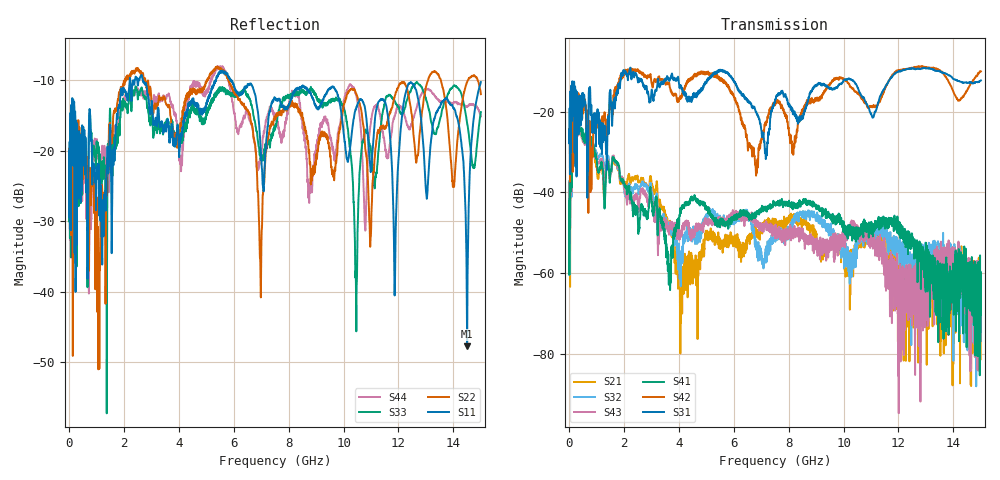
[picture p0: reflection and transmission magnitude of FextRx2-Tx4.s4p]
! FILE: N:\QM 2007\Prüfprotokolle\Highspeed\Konfektionierte Ltg\L45593-D106\D30\8216\0002\Fext\FextRx2-Tx4.s4p
# MHz S DB R 50.00
! FREQ  S11  S12  S13  S14
!  S21  S22  S23  S24
!  S31  S32  S33  S34
!  S41  S42  S43  S44
!  DB  ANG  DB  ANG  DB  ANG  DB  ANG
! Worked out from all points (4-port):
!   2999 points, 10 MHz to 15 GHz, reference 50 ohm
!   strongest paths, dB at 10 MHz, 3.755 GHz, 7.505 GHz, 11.26 GHz, 15 GHz:
!     S31: -24.6, -10.6, -17.4, -17.8, -12.3
!     S42: -24.3, -15.3, -18.5, -18.3, -10.1
!     S41: -42.2, -56.0, -42.7, -46.5, -70.3
!     S43: -48.5, -47.9, -48.9, -55.2, -64.2
!     S32: -41.6, -48.5, -49.1, -50.5, -67.4
!     S21: -49.6, -50.7, -47.5, -51.4, -69.8
!   lowest |S11| = -47.8 dB at 14.5 GHz (marker M1), VSWR 1.01, Z = 49.9 - j0.4 ohm
!   |S11| at or under -10 dB: start of sweep to 2.215 GHz; 2.693 GHz to 5.334 GHz (2.641 GHz wide, 65.8 % of centre); 5.923 GHz to end of sweep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
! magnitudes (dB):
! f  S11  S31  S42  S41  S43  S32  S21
! 10 MHz  -20.1  -24.6  -24.3  -42.2  -48.5  -41.6  -49.6
! 320 MHz  -26.8  -24.6  -19.0  -25.0  -25.6  -25.3  -25.5
! 4.11 GHz  -17.8  -14.4  -16.3  -44.0  -50.0  -55.1  -68.2
! 10.46 GHz  -14.1  -13.2  -15.1  -49.9  -49.1  -54.8  -53.0
! 12.47 GHz  -10.4  -9.4  -9.2  -51.1  -63.4  -64.0  -65.4
! 14.5 GHz  -47.8  -12.9  -14.8  -62.7  -67.7  -72.5  -57.3
! 15 GHz  -10.3  -12.3  -10.1  -70.3  -64.2  -67.4  -69.8
